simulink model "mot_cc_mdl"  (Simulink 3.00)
settings: Solver=ode45  StartTime=0.0  StopTime=10.0  RelTol=1e-6  AbsTol=1e-6
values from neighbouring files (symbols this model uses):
  b = Ic0*Ke/Wmax    (= 8.2054202412e-06)    [mot_cc_ss_int.m]    (also in mot_cc_ss_k.m; Regolatore_Rs_discreto.m = -h*alpha; mot_cc_ss.m)
  C0 = 0*N*m    (= 0)    [mot_cc_ss_int.m]    (also in mot_cc_ss_k.m; mot_cc_ss.m)
  Ia0 = 0    [mot_cc_ss_int.m]    (also in mot_cc_ss_k.m; mot_cc_ss.m)
  J = 9.2775e-006    (= 9.2775e-06)    [mot_cc_ss_int.m]    (also in mot_cc_ss_k.m; mot_cc_ss.m)
  Ke = Cmax/Imax    (= 0.00651965811966)    [mot_cc_ss_int.m]    (also in mot_cc_ss_k.m; mot_cc_ss.m)
  L = 60*10^-6    (= 6e-05)    [mot_cc_ss_int.m]    (also in mot_cc_ss_k.m; mot_cc_ss.m)
  R = Vn/Imax    (= 0.128205128205)    [mot_cc_ss_int.m]    (also in mot_cc_ss_k.m; mot_cc_ss.m)
  Tcsim = T_sim/1000    (= 8.42051458616e-06)    [mot_cc_ss_int.m]    (also in mot_cc_ss_k.m = 0.0001; mot_cc_ss.m = 0.001)
  Th0 = 0    [mot_cc_ss_int.m]    (also in mot_cc_ss_k.m; mot_cc_ss.m)
  V0 = 10*V    (= 10)    [mot_cc_ss.m]
  Wm0 = 0    [mot_cc_ss_int.m]    (also in mot_cc_ss_k.m; mot_cc_ss.m)
libraries: cstblocks x2

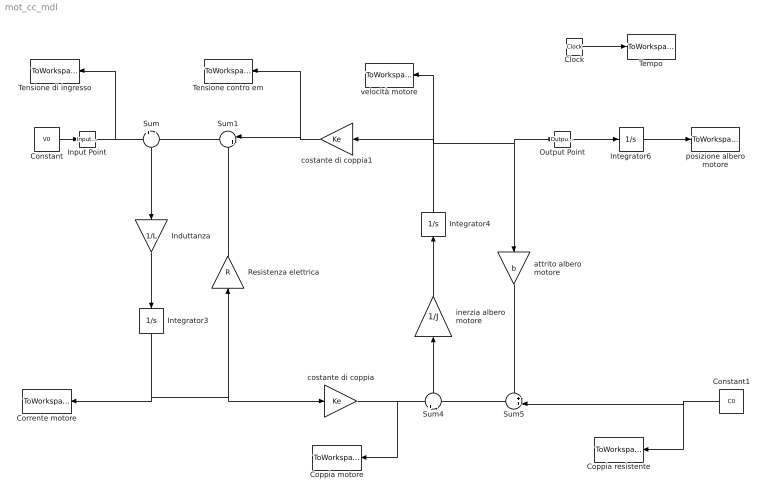
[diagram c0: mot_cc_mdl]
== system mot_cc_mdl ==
  Clock : Clock
  Constant : Constant  Value=V0
  Constant1 : Constant  Orientation=left  Value=C0
  Coppia motore : ToWorkspace  VariableName=Cm  SampleTime=Tcsim  SaveFormat=Matrix
  Coppia resistente : ToWorkspace  VariableName=Cr  SampleTime=Tcsim  SaveFormat=Matrix
  Corrente motore : ToWorkspace  VariableName=Ia  SampleTime=Tcsim  SaveFormat=Matrix
  Induttanza : Gain  Orientation=down  Gain=1/L  SaturateOnIntegerOverflow=on
  Input Point : cstblocks/Input Point  PerturbationValue=0
  Integrator3 : Integrator  Orientation=down  ExternalReset=none  InitialConditionSource=internal  InitialCondition=Ia0  LimitOutput=off  UpperSaturationLimit=inf  LowerSaturationLimit=-inf  ShowSaturationPort=off  ShowStatePort=off  AbsoluteTolerance=auto
  Integrator4 : Integrator  Orientation=up  ExternalReset=none  InitialConditionSource=internal  InitialCondition=Wm0  LimitOutput=off  UpperSaturationLimit=inf  LowerSaturationLimit=-inf  ShowSaturationPort=off  ShowStatePort=off  AbsoluteTolerance=auto
  Integrator6 : Integrator  ExternalReset=none  InitialConditionSource=internal  InitialCondition=Th0  LimitOutput=off  UpperSaturationLimit=inf  LowerSaturationLimit=-inf  ShowSaturationPort=off  ShowStatePort=off  AbsoluteTolerance=auto
  Output Point : cstblocks/Output Point  SigprobeOutputIndex=1
  Resistenza elettrica : Gain  Orientation=up  Gain=R  SaturateOnIntegerOverflow=on
  Sum : Sum  Orientation=down  Inputs=+|-  SaturateOnIntegerOverflow=on
  Sum1 : Sum  Orientation=left  Inputs=|++  SaturateOnIntegerOverflow=on
  Sum4 : Sum  Orientation=up  Inputs=+|-  SaturateOnIntegerOverflow=on
  Sum5 : Sum  Orientation=left  Inputs=++|  SaturateOnIntegerOverflow=on
  Tempo : ToWorkspace  VariableName=t  SampleTime=Tcsim  SaveFormat=Matrix
  Tensione contro em : ToWorkspace  VariableName=E  SampleTime=Tcsim  SaveFormat=Matrix
  Tensione di ingresso : ToWorkspace  VariableName=Vi  SampleTime=Tcsim  SaveFormat=Matrix
  attrito albero motore : Gain  Orientation=down  Gain=b  SaturateOnIntegerOverflow=on
  costante di coppia : Gain  Gain=Ke  SaturateOnIntegerOverflow=on
  costante di coppia1 : Gain  Orientation=left  Gain=Ke  SaturateOnIntegerOverflow=on
  inerzia albero motore : Gain  Orientation=up  Gain=1/J  SaturateOnIntegerOverflow=on
  posizione albero motore : ToWorkspace  VariableName=Th  SampleTime=Tcsim  SaveFormat=Matrix
  velocità motore : ToWorkspace  VariableName=Wm  SampleTime=Tcsim  SaveFormat=Matrix
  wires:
  Sum/1 -> Induttanza/1
  Induttanza/1 -> Integrator3/1
  Sum1/1 -> Sum/2
  Integrator3/1 -> Corrente motore/1, costante di coppia/1, Resistenza elettrica/1
  Resistenza elettrica/1 -> Sum1/2
  Sum4/1 -> inerzia albero motore/1
  inerzia albero motore/1 -> Integrator4/1
  Sum5/1 -> Sum4/2
  attrito albero motore/1 -> Sum5/1
  Constant1/1 -> Coppia resistente/1, Sum5/2
  Integrator4/1 -> velocità motore/1, costante di coppia1/1, attrito albero motore/1, Output Point/1
  Integrator6/1 -> posizione albero motore/1
  costante di coppia/1 -> Sum4/1, Coppia motore/1
  costante di coppia1/1 -> Sum1/1, Tensione contro em/1
  Clock/1 -> Tempo/1
  Constant/1 -> Input Point/1
  Input Point/1 -> Tensione di ingresso/1, Sum/1
  Output Point/1 -> Integrator6/1
